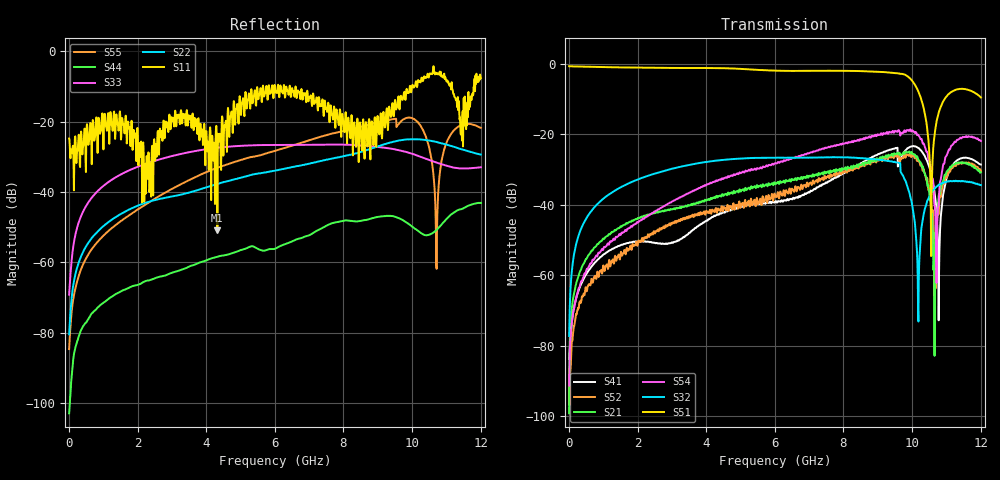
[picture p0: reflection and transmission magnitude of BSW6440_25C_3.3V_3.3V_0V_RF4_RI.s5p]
!	Test time	=	2022-08-08 18:13
!	Product	=	BSW6440
!	Temp	=	25C
!	VDD	=	3.3
!	Control_High	=	3.3
!	Control_Low	=	0
!	Logic	=	RF4
!	Porrt1	=	RFC
!	Porrt2	=	RF1
!	Porrt3	=	RF2
!	Porrt4	=	RF3
!	Porrt5	=	RF4
!	V1(LS)	=	3.3
!	V2(CTRL)	=	X
!	V3	=	X
!	V4	=	X
#	Hz	S	RI	R	50
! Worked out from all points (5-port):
!   1201 points, 5 MHz to 12.01 GHz, reference 50 ohm
!   strongest paths, dB at 5 MHz, 3.005 GHz, 6.005 GHz, 9.005 GHz, 12.01 GHz:
!     S51: -0.6, -1.1, -1.9, -2.2, -9.5
!     S32: -77.3, -29.8, -26.7, -27.2, -34.4
!     S54: -91.4, -39.1, -28.2, -20.1, -21.9
!     S21: -99.3, -41.3, -33.9, -27.2, -30.8
!     S52: -86.8, -45.4, -37.3, -27.3, -30.4
!     S41: -83.8, -50.7, -39.3, -25.7, -28.6
!   lowest |S11| = -50.9 dB at 4.325 GHz (marker M1), VSWR 1.01, Z = 50 + j0.283 ohm
!   |S11| at or under -10 dB: start of sweep to 5.652 GHz; 6.44 GHz to 9.934 GHz (3.494 GHz wide, 42.7 % of centre); 11.16 GHz to 11.81 GHz (645 MHz wide, 5.62 % of centre)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
